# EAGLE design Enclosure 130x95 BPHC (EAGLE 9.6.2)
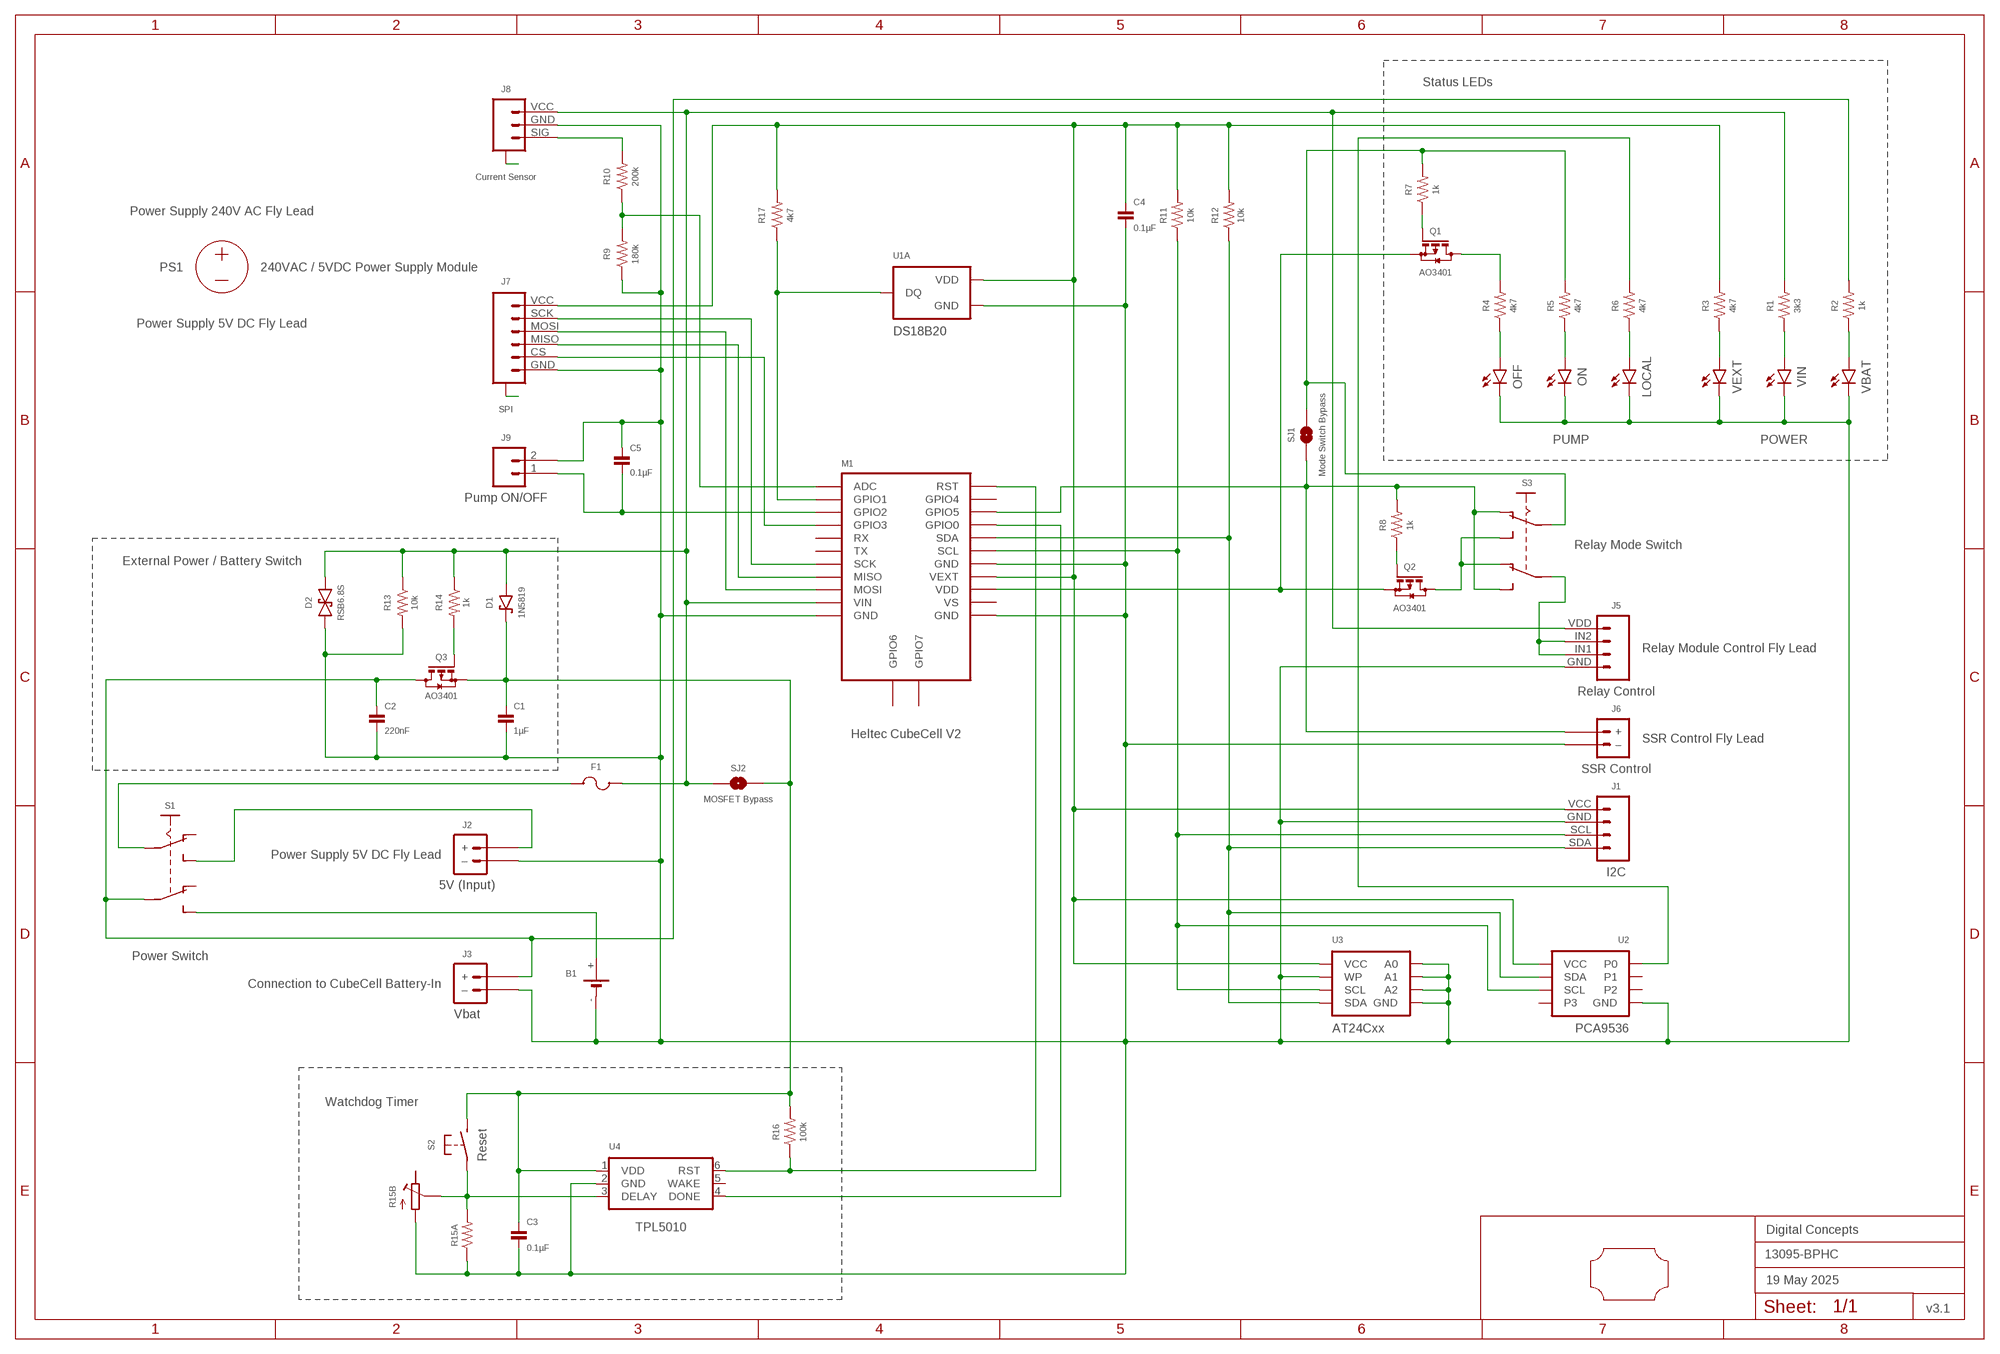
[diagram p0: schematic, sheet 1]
FRAME2 (A3L-LOC): DATE: 19 May 2025; OWNER: Digital Concepts; TITLE: 13095-BPHC; VERSION: v3.1

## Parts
B1  BATTERY-HOLDER-14500(AA)  [BATTERY-14500]
C1  1µF  CAPACITOR-0805  [C0805]
C2  220nF  CAPACITOR-0805  [C0805]
C3  0.1µF  CAPACITOR-0805  [C0805]
C4  0.1µF  CAPACITOR-0805  [C0805]
C5  0.1µF  CAPACITOR-0805  [C0805]
D1  1N5819  DIODE-SCHOTTKY-1N5819  [SOD-123]
D2  RSB6.8S  DIODE-SCHOTTKY-BIDIRECTIONAL  [VMD2]
F1  Fuse  MF-PSMF050X-2  [F0805]
J1  I2C  HEADER-1X4-I2C  [CONN_04-I2C]
J2  5V (Input)  JST-PH2.0-2-VERTICAL-POWER  [JST-PH2.0-2-VERTICAL-POWER]
J3  Vbat  JST-GH1.25-2-HORIZONTAL-POWER  [JST-GH1.25-2-HORIZONTAL]
J5  Relay Control  JST-PH2.0-4-HORIZONTAL-RELAY  [JST-PH2.0-4-HORIZONTAL-RELAY]
J6  SSR Control  JST-PH2.0-2-H-POWER  [JST-PH2.0-2-HORIZONTAL-POWER]
J7  SPI  JST-SH1.0-6-SMD-HORIZONTAL-SPI  [JST-SH1.0-6-HORIZONTAL-SPI]
J8  Current Sensor  JST-SH1.0-3-SMD-HORIZONTAL-SIG  [JST-SH1.0-3-HORIZONTAL-SIG]
J9  Pump ON/OFF  HEADER-1X2-GENERIC  [CONN_02-GENERIC]
LOCAL  LEDCHIP-LED0805  [CHIP-LED0805]
M1  Heltec CubeCell V2  HELTEC-CUBECELL  [HELTEC-CUBECELL]
OFF  LEDCHIP-LED0805  [CHIP-LED0805]
ON  LEDCHIP-LED0805  [CHIP-LED0805]
PCB1  PCB-OUTLINE-130X95-HALF-TOP  [PROTO-130X95-OUTLINE-HALF-TOP]
PS1  240VAC / 5VDC Power Supply Module  POWER_SUPPLY_MODULE  [AC_DC_POWER_SUPPLY]
Q1  AO3401  MOSFET-AO3401  [SOT-23]
Q2  AO3401  MOSFET-AO3401  [SOT-23]
Q3  AO3401  MOSFET-AO3401  [SOT-23]
R1  3k3  RESISTORR0805  [R0805]
R2  1k  RESISTORR0805  [R0805]
R3  4k7  RESISTORR0805  [R0805]
R4  4k7  RESISTORR0805  [R0805]
R5  4k7  RESISTORR0805  [R0805]
R6  4k7  RESISTORR0805  [R0805]
R7  1k  RESISTORR0805  [R0805]
R8  1k  RESISTORR0805  [R0805]
R9  180k  RESISTORR0805  [R0805]
R10  200k  RESISTORR0805  [R0805]
R11  10k  RESISTORR0805  [R0805]
R12  10k  RESISTORR0805  [R0805]
R13  10k  RESISTORR0805  [R0805]
R14  1k  RESISTORR0805  [R0805]
R15A  RESISTORR0805  [R0805]
R15B  RESISTOR-TRIMM-33  [RTRIM3*3]
R16  100k  RESISTORR0805  [R0805]
R17  4k7  RESISTORR0805  [R0805]
S1  Power Switch  SWITCH-SLIDE-DPDT-PTH  [SWITCH-DPDT-PTH]
S2  Reset  SWITCH-MOMENTARY-2-PIN  [SWITCH-2-PAD]
S3  Relay Mode Switch  SWITCH-SLIDE-DPDT-SMT  [SWITCH-DPDT-SMD]
SJ1  Mode Switch Bypass  SJ  [SJ]
SJ2  MOSFET Bypass  SJ  [SJ]
U1A  DS18B20  THERMOMETER-DS18B20  [TO-92]
U2  PCA9536  PCA9536-I2C-GPIO4  [SOP-8]
U3  AT24Cxx  AT24CXX-EEPROM  [SOP-8]
U4  TPL5010  TPL5010DDCR  [SOT-23-6]
VBAT  LEDCHIP-LED0805  [CHIP-LED0805]
VEXT  LEDCHIP-LED0805  [CHIP-LED0805]
VIN  LEDCHIP-LED0805  [CHIP-LED0805]

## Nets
A6: J8.A@1(A) J8.A@3(A)
A8: J7.A@1(A) J7.A@6(A)
GND: B1.- C1.2 C2.2 C3.2 C4.2 C5.1 D2.P$2 J1.GND J2.-(–) J3.-(–) J5.GND J6.-(–) J7.GND J8.GND J9.2 LOCAL.C M1.GND@11(GND) M1.GND@14(GND) M1.GND@18(GND) OFF.C ON.C R9.1 R13.2 R15A.1 R15B.1(A) U1A.1(GND) U2.4(GND) U3.1(A0) U3.2(A1) U3.3(A2) U3.4(GND) U3.7(WP) U4.2(GND) VBAT.C VEXT.C VIN.C
N$1: R6.2 U2.1(P0)
N$2: B1.+ S1.P$6(S2)
N$3: C5.2 J9.1 M1.GPIO2
N$4: C4.1 J1.VCC J7.VCC M1.VEXT R3.2 R11.2 R12.2 R17.2 U1A.3(VDD) U2.8(VCC) U3.8(VCC)
N$5: J1.SDA M1.SDA R12.1 U2.7(SDA) U3.5(SDA)
N$6: C1.1 C3.1 D1.C Q3.2(S) R16.2 S2.P$2(S) SJ2.2 U4.1(VDD)
N$7: J6.+ M1.GPIO5 R8.2 S3.P$1(O1) S3.P$6(S2) SJ1.1
N$8: M1.GPIO1 R17.1 U1A.2(DQ)
N$9: J1.SCL M1.SCL R11.1 U2.6(SCL) U3.6(SCL)
N$10: R2.1 VBAT.A
N$11: M1.GPIO0 U4.4(DONE)
N$12: OFF.A R4.1
N$13: R1.1 VIN.A
N$14: R3.1 VEXT.A
N$15: F1.2 S1.P$2(P1)
N$16: J2.+ S1.P$3(S1)
N$17: Q1.3(D) R4.2
N$18: M1.ADC R9.2 R10.1
N$19: ON.A R5.1
N$20: LOCAL.A R6.1
N$21: D1.A D2.P$1 F1.1 J5.VDD J8.VCC M1.VIN R1.2 R13.1 R14.1 SJ2.1
N$22: Q1.1(G) R7.1
N$23: Q2.3(D) S3.P$3(S1) S3.P$4(O2)
N$24: Q2.1(G) R8.1
N$25: J8.SIG R10.2
N$26: R5.2 R7.2 S3.P$2(P1) SJ1.2
N$27: J5.IN1 J5.IN2 S3.P$5(P2)
N$28: J7.SCK M1.SCK
N$29: J7.MOSI M1.MOSI
N$30: J7.MISO M1.MISO
N$31: J7.CS M1.GPIO3
N$34: C2.1 J3.+ Q3.3(D) R2.2 S1.P$5(P2)
N$36: R15A.2 R15B.2(S) S2.P$1(P) U4.3(DELAY)
N$37: M1.RST R16.1 U4.6(RST)
N$43: Q3.1(G) R14.2
VCC: M1.VDD Q1.2(S) Q2.2(S)
Unconnected: M1.GPIO4 M1.GPIO6 M1.GPIO7 M1.RX M1.TX M1.VS R15B.3(E) S1.P$1(O1) S1.P$4(O2) U2.2(P1) U2.3(P2) U2.5(P3) U4.5(WAKE)

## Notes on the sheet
- Status LEDs
- Power Supply 240V AC Fly Lead
- Power Supply 5V DC Fly Lead
- PUMP | POWER
- External Power / Battery Switch
- Relay Module Control Fly Lead
- SSR Control Fly Lead
- Power Supply 5V DC Fly Lead
- Connection to CubeCell Battery-In
- Watchdog Timer

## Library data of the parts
B1 = digitalconcepts:BATTERY-HOLDER-14500(AA): 14500 (AA) battery holder
C1-C5 = digitalconcepts:CAPACITOR-0805: 0805 Capacitor
D1 = digitalconcepts:DIODE-SCHOTTKY-1N5819: 1N5819 Schottky Diode SOD-123
D2 = digitalconcepts:DIODE-SCHOTTKY-BIDIRECTIONAL: Schottky Bidirectional Diode
F1 = digitalconcepts:MF-PSMF050X-2: PTC Resettable Fuse
J1 = digitalconcepts:HEADER-1X4-I2C: I2C Interface [Pin 1 Vcc] 4-Pin Header
J2 = digitalconcepts:JST-PH2.0-2-VERTICAL-POWER: JST PH2.0 2P PTH Connector (Power)
J3 = digitalconcepts:JST-GH1.25-2-HORIZONTAL-POWER: JST GH1.25 2P PTH Connector (Power)
J5 = digitalconcepts:JST-PH2.0-4-HORIZONTAL-RELAY: PH2.0 4P Horizontal Connector with Relay Labels
J6 = digitalconcepts:JST-PH2.0-2-H-POWER: PH2.0 2P Right Angle Connector with power pin labelling
J7 = digitalconcepts:JST-SH1.0-6-SMD-HORIZONTAL-SPI: JST SH1.0 6P SMD SPI horizontal connector
J8 = digitalconcepts:JST-SH1.0-3-SMD-HORIZONTAL-SIG: JST SH1.0 3P SMD Horizontal Connector with Signal
J9 = digitalconcepts:HEADER-1X2-GENERIC: Single Row 2-Pin Header
LOCAL OFF ON VBAT VEXT VIN = digitalconcepts:LED: LED
M1 = digitalconcepts:HELTEC-CUBECELL: Heltec CubeCell Development Board
PCB1 = digitalconcepts:PCB-OUTLINE-130X95-HALF-TOP: PCB half (sandwich top) enclosure (75 x 95) outline for 130 x 95 enclosure
PS1 = digitalconcepts:POWER_SUPPLY_MODULE: AC/DC Power Supply Module
Q1-Q3 = digitalconcepts:MOSFET-AO3401: AO3401 P-Channel MOSFET
R1-R14 R15A R16 R17 = digitalconcepts:RESISTOR: Resistor; SPICEPREFIX: R
R15B = digitalconcepts:RESISTOR-TRIMM-3*3: Trimm Resistor - 3*3 SMD
S1 = digitalconcepts:SWITCH-SLIDE-DPDT-PTH: Switch DPDT PTH
S2 = digitalconcepts:SWITCH-MOMENTARY-2-PIN: 2 Pin Momentary Switch
S3 = digitalconcepts:SWITCH-SLIDE-DPDT-SMT: Switch DPDT SMT
SJ1 SJ2 = digitalconcepts:SJ: Solder Jumper
U1A = digitalconcepts:THERMOMETER-DS18B20: Digital Thermometer -55C-125C TO92-3; AVAILABILITY: Bad; DESCRIPTION: Temperature Sensor Digital, Local -55°C ~ 125°C 12 b 8-uMAX; MF: Maxim Integrated; MP: DS18B20; PACKAGE: TO-92 Maxim Integrated; PRICE: None
U2 = digitalconcepts:PCA9536-I2C-GPIO4: PCA9536 4-bit I2C GPIO Expander
U3 = digitalconcepts:AT24CXX-EEPROM: AT24Cxx EEPROM SOP-8
U4 = digitalconcepts:TPL5010DDCR: TPL5010 Nano-Power System Timer with Watchdog

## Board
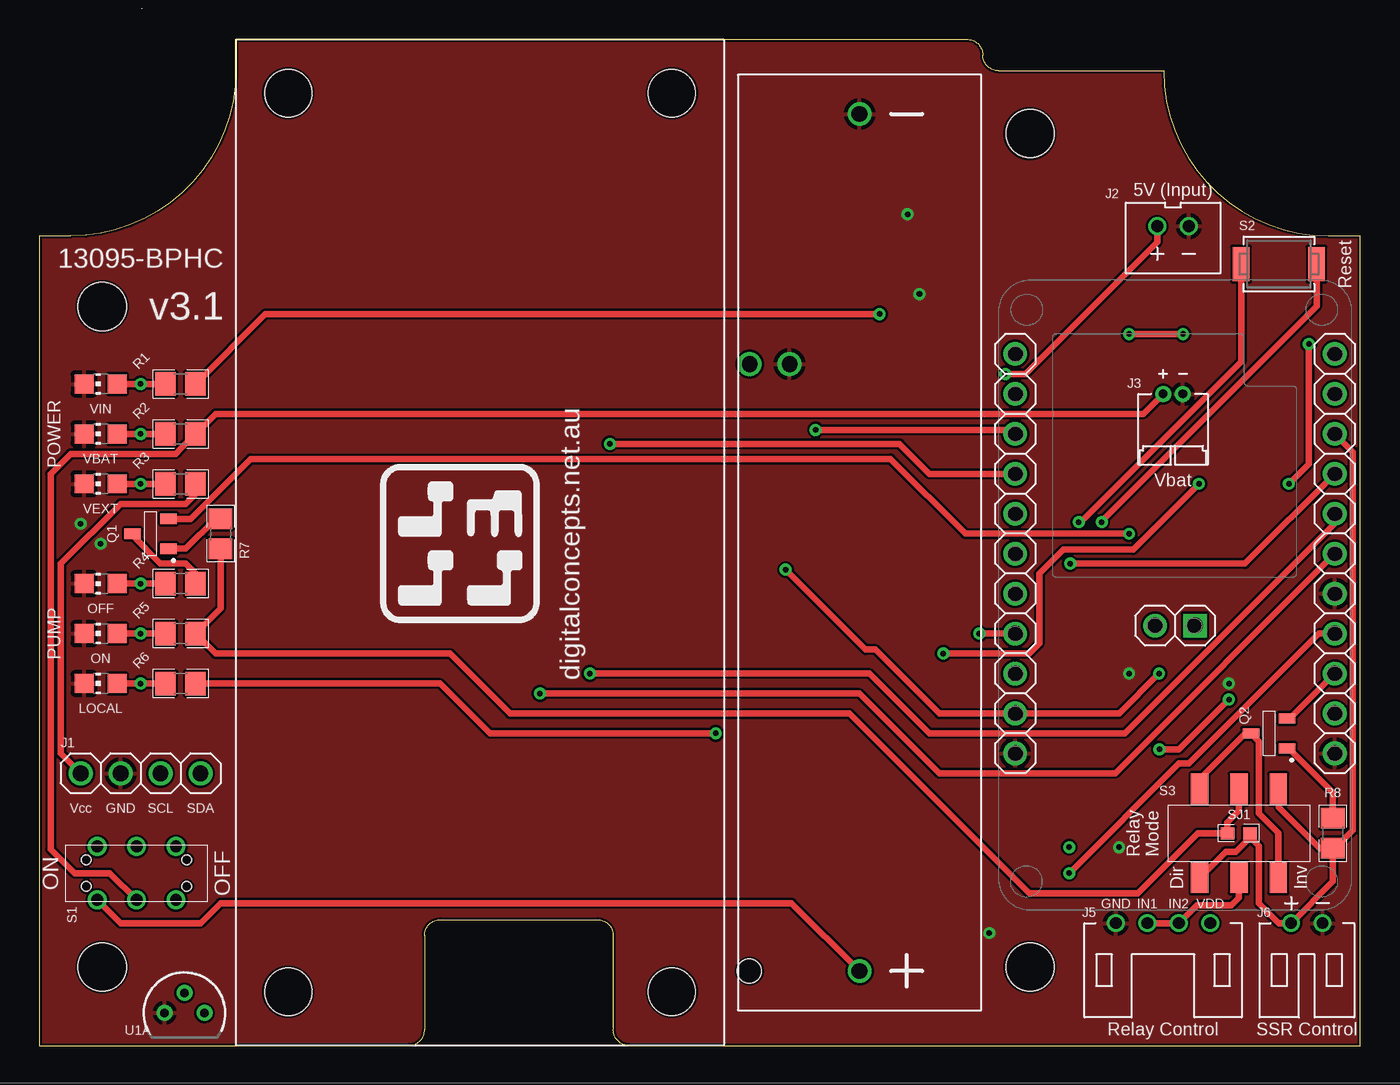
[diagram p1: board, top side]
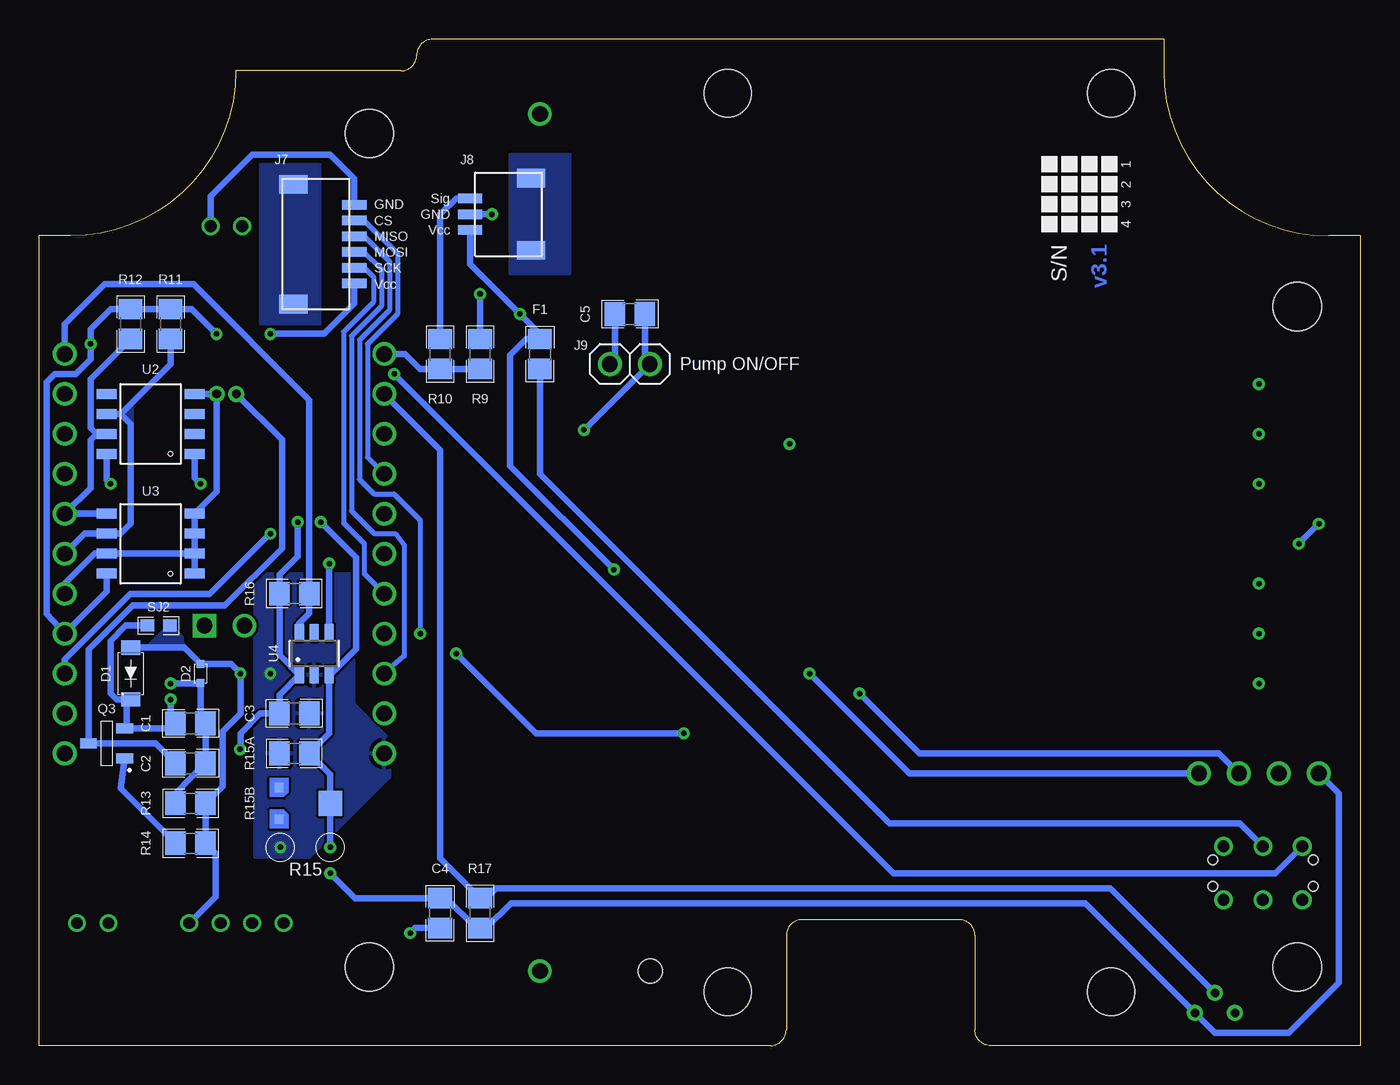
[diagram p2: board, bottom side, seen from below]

Size 84 x 64 mm. Coordinates in mm from the lower left corner, seen from the top.
Copper layers (1*16): Top 0.035mm / dielectric 1.5mm / Bottom 0.035mm
Design rules "default *": minimum track width 6mil, minimum drill 0.35mm, track to track 6mil, track to pad 6mil, pad to pad 6mil, via to via 6mil, smd to smd 6mil, copper to edge 6mil, drill to drill 6mil, minimum pad ring 1mil, minimum via ring 8mil, stop-mask expansion 4mil, vias tented up to drill 0mil, thermal gap 10mil

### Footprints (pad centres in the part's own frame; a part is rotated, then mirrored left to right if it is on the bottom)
BATTERY-14500 = drill 1: + -27.25,0; - 27.25,0 | hole 1.524: -27.25,7
C0805 = smd 1.3 x 1.5: 1 -0.95,0; 2 0.95,0
SOD-123 = smd 0.91 x 1.22: A -1.65,0; C 1.65,0
VMD2 = smd 0.5 x 0.5: P$1 -0.6,0; P$2 0.6,0
F0805 = smd 1.3 x 1.5: 1 -0.95,0; 2 0.95,0
CONN_04-I2C = drill 1 pad 1.524: GND 2.54,0; SCL 5.08,0; SDA 7.62,0; VCC 0,0
JST-PH2.0-2-VERTICAL-POWER = drill 0.75: + -1,0; - 1,0
JST-GH1.25-2-HORIZONTAL = drill 0.55 pad 1.016: + -0.625,0; - 0.625,0
JST-PH2.0-4-HORIZONTAL-RELAY = drill 0.75: GND 3,0; IN1 1,0; IN2 -1,0; VDD -3,0
JST-PH2.0-2-HORIZONTAL-POWER = drill 0.75: + 1,0; - -1,0
JST-SH1.0-6-HORIZONTAL-SPI = smd 1.2 x 1.8: A@1 -3.8,-1.335; A@6 3.8,-1.335 | smd 0.6 x 1.55: CS -1.5,2.54; GND -2.5,2.54; MISO -0.5,2.54; MOSI 0.5,2.54; SCK 1.5,2.54; VCC 2.5,2.54
JST-SH1.0-3-HORIZONTAL-SIG = smd 1.2 x 1.8: A@1 -2.3,-1.335; A@3 2.3,-1.335 | smd 0.6 x 1.55: GND 0,2.54; SIG 1,2.54; VCC -1,2.54
CONN_02-GENERIC = drill 1 pad 1.524: 1 0,0; 2 2.54,0
CHIP-LED0805 = smd 1.2 x 1.2: A 0,-1.05; C 0,1.05
HELTEC-CUBECELL = drill 1: ADC 0,0; GND@11 0,25.4; GND@14 -20.32,25.4; GND@18 -20.32,15.24; GPIO0 -20.32,7.62; GPIO1 0,2.54; GPIO2 0,5.08; GPIO3 0,7.62; GPIO4 -20.32,2.54; GPIO5 -20.32,5.08; GPIO6 -8.89,17.272; MISO 0,17.78; MOSI 0,20.32; RST -20.32,0; RX 0,10.16; SCK 0,15.24; SCL -20.32,12.7; SDA -20.32,10.16; TX 0,12.7; VDD -20.32,20.32; VEXT -20.32,17.78; VIN 0,22.86; VS -20.32,22.86 | drill 1 square: GPIO7 -11.43,17.272
PROTO-130X95-OUTLINE-HALF-TOP = hole 3.048: -38,10; 21,21; 21,-32; -38,-32
AC_DC_POWER_SUPPLY = hole 3: -28.575,12.192; -28.575,-12.192; 28.575,-12.192; 28.575,12.192
SOT-23 = smd 0.65 x 1.05: 1 -0.95,-1.15; 2 0.95,-1.15; 3 0,1.15
R0805 = smd 1.3 x 1.5: 1 -0.95,0; 2 0.95,0
RTRIM3*3 = smd 0.6 x 0.6: 1 -1,-1.6; 3 1,-1.6 | smd 1.6 x 1.5: 2 0,1.65
SWITCH-DPDT-PTH = drill 0.75 pad 1.19: P$1 -1.7,2.5; P$2 -1.7,0; P$3 -1.7,-2.5; P$4 1.7,2.5; P$5 1.7,0; P$6 1.7,-2.5 | hole 0.6: 0.85,3.2; -0.85,3.2; 0.85,-3.2; -0.85,-3.2
SWITCH-2-PAD = smd 1.067 x 2.184: P$1 -2.4,0; P$2 2.4,0
SWITCH-DPDT-SMD = smd 1.95 x 1.1: P$1 -2.825,2.5; P$2 -2.825,0; P$3 -2.825,-2.5; P$4 2.825,2.5; P$5 2.825,0; P$6 2.825,-2.5
SJ = smd 0.864 x 0.762: 1 -0.711,0; 2 0.711,0
TO-92 = drill 0.55 pad 1.016: 1 -1.27,0; 2 0,1.27; 3 1.27,0
SOP-8 = smd 0.635 x 1.27: 1 -1.905,-2.794; 2 -0.635,-2.794; 3 0.635,-2.794; 4 1.905,-2.794; 5 1.905,2.794; 6 0.635,2.794; 7 -0.635,2.794; 8 -1.905,2.794
SOT-23-6 = smd 1.1 x 0.6: 1 -1.35,0.95; 2 -1.35,0; 3 -1.35,-0.95; 4 1.35,-0.95; 5 1.35,0; 6 1.35,0.95

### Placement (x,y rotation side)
B1  52.16,32 90 top
C1  74.39,20.49 0 bottom
C2  74.39,17.95 0 bottom
C3  67.78,21.13 0 bottom
C4  58.51,8.43 270 bottom
C5  46.45,46.53 0 bottom
D1  78.19,23.67 270 bottom
D2  73.75,23.67 270 bottom
F1  52.16,43.98 270 bottom
J1  2.63,17.32 0 top
J2  72.1,52.11 0 top
J3  72.1,41.45 0 top
J5  71.46,7.79 180 top
J6  80.61,7.79 180 top
J7  66.51,50.97 270 bottom
J8  54.06,52.88 90 bottom
J9  45.17,43.35 180 bottom
LOCAL  3.9,23.03 90 top
M1  62.07,43.98 180 top
OFF  3.9,29.38 90 top
ON  3.9,26.21 90 top
PCB1  42,37 0 top
PS1  28.03,32 90 top
Q1  7.07,32.55 90 top
Q2  78.19,19.86 90 top
Q3  79.72,19.22 90 bottom
R1  8.98,42.08 0 top
R2  8.98,38.91 0 top
R3  8.98,35.73 0 top
R4  8.98,29.38 0 top
R5  8.98,26.21 0 top
R6  8.98,23.03 0 top
R7  11.52,32.55 270 top
R8  82.26,13.51 270 top
R9  55.97,43.98 270 bottom
R10  58.51,43.98 90 bottom
R11  75.66,45.89 90 bottom
R12  78.19,45.89 90 bottom
R13  74.39,15.41 180 bottom
R14  74.39,12.87 180 bottom
R15A  67.78,18.59 0 bottom
R15B  67.15,15.41 270 bottom
R16  67.78,28.75 180 bottom
R17  55.97,8.43 270 bottom
S1  6.19,10.97 270 top
S2  78.83,49.7 0 top
S3  76.29,13.51 270 top
SJ1  76.29,13.51 180 top
SJ2  76.42,26.71 180 bottom
U1A  9.23,2.08 0 top
U2  76.92,39.54 90 bottom
U3  76.92,31.92 90 bottom
U4  66.51,24.94 90 bottom
VBAT  3.9,38.91 90 top
VEXT  3.9,35.73 90 top
VIN  3.9,42.08 90 top

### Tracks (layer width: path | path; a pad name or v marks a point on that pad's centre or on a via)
A6
  pour Bottom (no thermals): 50.25,56.69 54.06,56.69 54.06,49.07 50.25,49.07
A8
  pour Bottom (no thermals): 69.94,56.05 69.94,45.89 66.13,45.89 66.13,56.05
GND  (via drill 0.35)
  Bottom 0.406: R13.2 75.33,16.05 74.33,17.05 74.33,17.06 C2.2 C1.2 73.75,20.81 D2.P$2 73.78,23.03 v75.66,23.03 | U3.2 U3.3 U3.4 72.72,35.23 J3.- U2.4 | U3.2 U3.1 | U3.2 U3.7 80.48,31.29 82.39,29.38 M1.GND@18 | v60.41,7.16 60.09,7.48 C4.2 | v2.63,33.19 v3.9,31.92 | C5.1 47.39,43.67 J9.2 | J2.- 73.1,54.02 70.46,56.65 65.5,56.65 63.97,55.12 J7.GND | v55.21,52.88 J8.GND | R9.1 v55.97,47.8
  other vias: 68.67,12.62 69.3,23.67
  pour Top (rank 5): -1.18,64.94 -1.18,-1.1 85.18,-1.1 85.18,64.94
  pour Bottom (rank 2): 70.32,30.02 70.32,11.98 66.77,11.98 61.69,17.06 61.69,19.47 63.97,21.76 63.97,30.02
  pour Bottom: 73.75,23.03 74.39,23.03 73.75,22.4
N$1  (via drill 0.35)
  Top 0.406: v43.02,19.86 28.66,19.86 25.49,23.03 R6.2 | v73.75,35.73 69.56,31.54 65.11,31.54 63.59,30.02 63.59,25.57 62.95,24.94 v57.49,24.94
  Bottom 0.406: U2.1 74.13,36.11 v73.75,35.73 | v57.49,24.94 52.41,19.86 v43.02,19.86
N$2
  Top 0.406: B1.+ 47.85,9.06 11.52,9.06 10.25,7.79 5.16,7.79 S1.P$6
N$3  (via drill 0.35)
  Top 0.406: M1.GPIO2 61.81,39.16 v49.37,39.16
  Bottom 0.406: v49.37,39.16 J9.1 45.49,43.67 C5.2
N$4  (via drill 0.35)
  Top 0.406: R3.2 9.93,35.09 9.3,34.46 5.17,34.46 1.36,30.65 1.36,18.59 J1.VCC | v80.73,44.62 80.73,37 v79.47,35.73 | v72.73,45.26 v69.3,45.26 | M1.VEXT 81.37,26.21 73.11,17.95 72.48,17.95 v65.5,10.97
  Bottom 0.406: U3.8 79.72,28.87 M1.VEXT 83.53,27.46 83.53,42.21 83.02,42.72 81.69,42.72 80.73,43.67 v80.73,44.62 80.73,45.57 79.47,46.84 R12.2 R11.2 74.32,46.84 v72.73,45.26 | v65.5,10.97 63.91,9.38 C4.1 58.13,9.38 56.23,7.48 R17.2 55.59,7.48 54,9.06 17.49,9.06 U1A.3 9.23,0.81 4.53,0.81 1.36,3.98 1.36,16.05 J1.VCC | U2.8 79.72,35.98 v79.47,35.73 | v69.3,45.26 68.94,45.3 65.88,45.3 63.97,47.2 J7.VCC
N$5  (via drill 0.35)
  Top 0.406: M1.SDA 82.39,33.22 69.02,19.86 56.61,19.86 52.8,23.67 v35.02,23.67
  Bottom 0.406: v35.02,23.67 28.66,17.32 J1.SDA | U3.5 M1.SDA 80.73,35.48 80.73,38.52 80.35,38.91 | 80.35,38.91 80.73,39.29 80.73,42.4 R12.1 | U2.7 80.35,38.91
N$6  (via drill 0.35)
  Top 0.406: v71.24,18.84 72.48,18.84 v75.66,22.01 | S2.P$2 81.23,47.02 67.56,33.36 v67.56,33.29
  Bottom 0.406: v75.66,22.01 75.66,20.81 C1.1 75.66,20.17 Q3.2 78.44,20.3 78.44,21.77 D1.C 79.08,22.02 79.47,22.4 79.47,25.74 78.49,26.71 SJ2.2 | v71.24,18.84 71.21,18.84 71.21,19.86 69.94,21.13 C3.1 68.73,22.32 U4.1 68.73,24.86 R16.2 68.73,29.95 67.56,31.12 v67.56,33.29
N$7
  Top 0.406: M1.GPIO5 83.53,37.76 83.53,13.7 82.39,12.56 R8.2 | S3.P$1 78.83,16.29 78.83,15.16 81.43,12.56 R8.2 | R8.2 82.26,10.44 J6.+ 78.83,7.79 77.56,9.06 77.56,12.69 77,13.25 SJ1.1 77,13.26 76.08,12.33 75.44,12.33 S3.P$6
N$8
  Bottom 0.406: U1A.2 15.9,10.01 54.95,10.01 55.59,9.38 R17.1 58.51,11.92 58.51,37.89 M1.GPIO1
N$9  (via drill 0.35)
  Top 0.406: M1.SCL 68.42,17.32 57.24,17.32 52.16,22.4 v31.84,22.4
  Bottom 0.406: M1.SCL 81.12,32.55 U3.6 78.83,32.55 78.19,33.19 78.19,39.54 78.83,40.18 | v31.84,22.4 28.03,18.59 8.98,18.59 J1.SCL | U2.6 78.83,40.18 | R11.1 75.66,43.35 78.83,40.18
  pour Bottom: 78.83,40.18 78.19,40.81 78.19,39.54
N$10  (via drill 0.35)
  Top 0.406: VBAT.A v6.44,38.91 R2.1
N$11  (via drill 0.35)
  Top 0.406: M1.GPIO0 76.67,30.65 v65.56,30.65
  Bottom 0.406: v65.56,30.65 U4.4
N$12  (via drill 0.35)
  Top 0.406: R4.1 v6.44,29.38 OFF.A
N$13  (via drill 0.35)
  Top 0.406: VIN.A v6.44,42.08 R1.1
N$14  (via drill 0.35)
  Top 0.406: R3.1 v6.44,35.73 VEXT.A
N$15
  Bottom 0.406: F1.2 52.16,36.37 29.94,14.14 7.66,14.14 S1.P$2
N$16  (via drill 0.35)
  Top 0.406: J2.+ 71.1,51.1 62.72,42.72 v61.43,42.72
  Bottom 0.406: v61.43,42.72 29.68,10.97 5.39,10.97 S1.P$3
N$17
  Top 0.406: R4.2 9.93,30.02 9.29,30.65 7.7,30.65 5.92,32.43 Q1.3
N$18
  Bottom 0.406: R9.2 R10.1 59.78,43.04 60.73,43.98 M1.ADC
N$19  (via drill 0.35)
  Top 0.406: R5.1 v6.44,26.21 ON.A
N$20  (via drill 0.35)
  Top 0.406: LOCAL.A v6.44,23.03 R6.1
N$21  (via drill 0.35)
  Top 0.406: v53.43,46.53 14.38,46.53 R1.2 | v47.46,30.27 52.54,25.19 53.18,25.19 57.24,21.13 M1.VIN 68.67,21.13 v71.21,23.67
  Bottom 0.406: D1.A 74.8,25.32 D2.P$1 71.81,24.27 v71.21,23.67 71.21,21.13 72.35,19.98 72.35,16.49 R13.1 R14.1 72.8,12.24 72.8,9.45 J5.VDD | v47.46,30.27 54.06,36.87 54.06,43.92 53.05,44.94 F1.1 52.16,45.26 v53.43,46.53 56.61,49.7 J8.VCC
  pour Bottom (no thermals): 74.8,25.32 75.02,25.57 75.02,25.95 75.4,26.33 76.04,26.33 77.05,25.32
N$22
  Top 0.406: Q1.1 9.3,31.61 11.2,33.51 R7.1
N$23
  Top 0.406: S3.P$4 78.79,13.55 77.55,14.78 77.55,19.35 Q2.3 76.68,19.86 73.79,16.97 S3.P$3
N$24
  Top 0.406: R8.1 82.26,16.11 79.47,18.91 Q2.1
N$25
  Bottom 0.406: J8.SIG 57.51,53.88 58.51,52.88 R10.2
N$26
  Top 0.406: R7.2 11.52,27.8 R5.2 11.2,24.94 26.12,24.94 29.94,21.13 51.52,21.13 62.95,9.7 69.86,9.7 73.67,13.51 SJ1.2 75.55,13.54 75.55,14.19 76.29,14.93 S3.P$2
N$27
  Top 0.406: J5.IN1 J5.IN2 73.61,8.93 75.81,8.93 76.29,9.41 S3.P$5
N$28
  Bottom 0.305: J7.SCK 63.34,49.47 62.75,48.89 62.75,47.29 64.66,45.38 64.66,33.24 63.34,31.92 63.34,30.02 M1.SCK
N$29
  Bottom 0.305: J7.MOSI 63.34,50.47 62.24,49.38 62.24,47.03 64.15,45.13 64.15,34 62.7,32.55 61.36,32.55 60.8,31.84 60.8,24.77 M1.MOSI
N$30  (via drill 0.35)
  Top 0.406: M1.MISO v59.78,26.21
  Bottom 0.305: J7.MISO 63.34,51.47 61.74,49.87 61.74,46.78 63.64,44.87 63.64,36.01 62.71,35.08 61.44,35.08 59.78,33.42 v59.78,26.21
N$31  (via drill 0.35)
  Top 0.406: v36.28,38.27 54.7,38.27 56.61,36.37 M1.GPIO3
  Bottom 0.305: M1.GPIO3 63.13,37.43 63.13,44.62 61.23,46.53 61.23,50.36 63.34,52.47 J7.CS
N$34
  Top 0.406: S1.P$5 4.49,10.97 2.25,10.97 0.72,12.49 0.72,36.37 1.99,37.64 8.66,37.64 9.04,38.01 R2.2 11.2,40.18 70.2,40.18 J3.+
  Bottom 0.406: C2.1 76.61,19.22 Q3.3 80.87,25.18 78.07,27.98 72.2,27.98 68.57,31.62 68.57,38.54 J3.+
N$36  (via drill 0.35)
  Top 0.406: S2.P$1 76.43,43.49 66.13,33.19 66.1,33.22 v66.1,33.29
  Bottom 0.406: v65.5,12.62 R15B.2 65.5,17.25 R15A.2 65.56,19.86 U4.3 65.5,23.59 63.84,25.24 63.84,31.04 v66.1,33.29
N$37
  Bottom 0.406: M1.RST 82.39,45.89 79.85,48.43 74.2,48.43 66.83,41.06 R16.1 66.83,27.48 67.46,26.85 U4.6
N$43
  Bottom 0.406: R14.2 78.82,16.36 Q3.1
VCC  (via drill 0.35)
  Top 0.406: v69.3,32.55 58.89,32.55 54.13,37.32 13.42,37.32 9.61,33.51 Q1.2 | M1.VDD 79.53,20.81 Q2.2
  Bottom 0.406: v69.3,32.55 73.15,28.71 78.23,28.71 82.39,24.55 M1.VDD

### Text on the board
Bottom: v3.1
tPlace: 13095-BPHC | digitalconcepts.net.au
bPlace: 1 | 2 | 3 | 4 | S/N
tNames: v3.1 | POWER | PUMP | Vcc | GND | SCL | SDA | Relay / Mode | ON | OFF | Dir | Inv
bNames: Sig | GND | GND | CS | Vcc | MISO | MOSI | SCK | Vcc | R15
